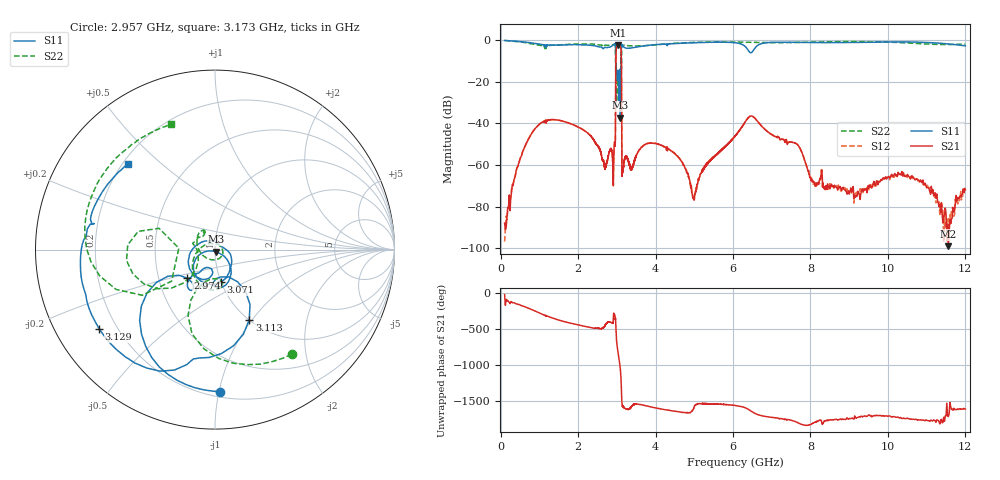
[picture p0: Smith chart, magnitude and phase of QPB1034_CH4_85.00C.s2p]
! TDS: k:\Engsetup\Winsaw\QPB1034_ALL
! Channel 1
! Ports=1 2
! seg 1=100.000000 1100.000000 51
! seg 2=1101.000000 1301.000000 201
! seg 3=1302.000000 2302.000000 101
! seg 4=2303.000000 3503.000000 1201
! seg 5=3504.000000 5204.000000 171
! seg 6=5205.000000 6405.000000 1201
! seg 7=6406.000000 8506.000000 211
! seg 8=8507.000000 12007.000000 176
! Points=3313
! FailCode=0
! Topology=ALL_SE(12)
!VNA Cal loaded =QPB1034_ALL_85C
!PS1(V)= 5.000
!PS(mA)= 0.444
!PS2(V)= 1.170
!PS(mA)= -0.001
!PS3(V)= 0.630
!PS(mA)= -0.002
!PS4(V)= 0.630
!PS(mA)= -0.003
!Temp (C)= 85.00
# MHz S DB R 50
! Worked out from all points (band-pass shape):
!   3313 points, 100 MHz to 12.01 GHz, reference 50 ohm
!   highest |S21| = -2.66 dB at 3.027 GHz (marker M1); lowest = -98.9 dB at 11.57 GHz (marker M2)
!   |S21| within 3 dB of the highest: 2.981 GHz to 3.111 GHz (129.4 MHz wide, 4.25 % of centre)
!   lowest |S11| = -37.4 dB at 3.092 GHz (marker M3), VSWR 1.03, Z = 50.7 - j1.18 ohm
!   |S11| at or under -10 dB: 2.972 GHz to 3.111 GHz (139.6 MHz wide, 4.59 % of centre)
!   |S22| runs from -29.9 to -0.3 dB; largest |S21 - S12| = 0.0043
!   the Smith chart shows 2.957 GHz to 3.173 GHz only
!   S11 on the Smith chart (normalised r, x): 2.957 GHz: 0.24, -1.00; 2.974 GHz: 0.70, -0.23; 3.071 GHz: 1.00, -0.38; 3.113 GHz: 1.01, -0.97; 3.129 GHz: 0.13, -0.30; 3.173 GHz: 0.22, +0.39
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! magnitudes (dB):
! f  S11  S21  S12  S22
! 100 MHz  -0.3  -87.8  -96.7  -0.3
! 240 MHz  -0.5  -81.9  -76.4  -0.5
! 500 MHz  -0.9  -57.0  -56.9  -1.0
! 1.1 GHz  -2.4  -39.2  -39.2  -2.8
! 2.434 GHz  -2.9  -49.1  -49.0  -2.1
! 2.905 GHz  -2.5  -67.9  -67.9  -2.3
! 2.957 GHz  -2.0  -51.0  -51.0  -2.8
! 2.974 GHz  -13.1  -10.2  -10.2  -14.2
! 3.027 GHz  -14.6  -2.7  -2.7  -19.5
! 3.071 GHz  -14.7  -3.1  -3.1  -19.2
! 3.092 GHz  -37.4  -3.4  -3.4  -18.7
! 3.113 GHz  -7.2  -7.2  -7.1  -7.1
! 3.129 GHz  -2.1  -53.9  -53.9  -2.6
! 3.144 GHz  -2.7  -60.8  -60.7  -2.5
! 3.173 GHz  -3.4  -60.2  -60.3  -2.6
! 4.044 GHz  -2.3  -49.9  -49.9  -2.3
! 5.014 GHz  -1.4  -73.8  -74.4  -1.2
! 5.406 GHz  -1.2  -58.1  -58.0  -1.1
! 6.456 GHz  -6.2  -36.6  -36.6  -1.2
! 8.106 GHz  -1.3  -68.3  -69.1  -1.1
! 11.57 GHz  -2.0  -98.9  -85.8  -2.3
! 12.01 GHz  -2.9  -71.9  -71.9  -2.0
